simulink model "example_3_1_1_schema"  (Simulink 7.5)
settings: Solver=ode45  StartTime=0.0  StopTime=100  FixedStep=0.001  RelTol=1e-3
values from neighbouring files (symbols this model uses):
  A = [-.4 0 -0.01; 1 0 0; -1.4 9.8 -0.02]    [example_3_1_1_podklad.m]
  AA = A-B*K    [example_3_1_1_podklad.m]
  AAd = Ad-Bd*Kd    [example_3_1_1_podklad.m]
  B = [6.3;0;9.8]    [example_3_1_1_podklad.m]
  C = [0 0 1]    [example_3_1_1_podklad.m]
  D = 0    [example_3_1_1_podklad.m]
  I = eye(m,n)    [example_3_1_1_podklad.m]
  Ng = lqr_kompenzace(A,B,C,D,K)    [example_3_1_1_podklad.m]    (also in lqr_kompenzace.m = Nu + K*Nx)
  T = 0.1    [example_3_1_1_podklad.m]
undefined symbols (not defined in the file or in its folder): Ad, Bd, Cd, Dd, K, Kd

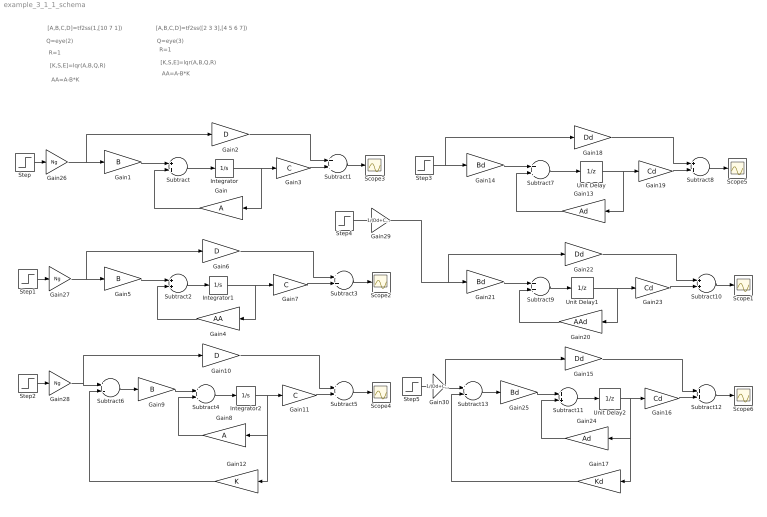
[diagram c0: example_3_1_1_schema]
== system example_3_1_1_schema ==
  note: [A,B,C,D]=tf2ss(1,[10 7 1])
  note: [K,S,E]=lqr(A,B,Q,R)
  note: Q=eye(2)
  note: R=1
  note: [K,S,E]=lqr(A,B,Q,R)
  note: Q=eye(3)
  note: R=1
  note: AA=A-B*K
  note: AA=A-B*K
  note: [A,B,C,D]=tf2ss([2 3 3],[4 5 6 7])
  Gain : Gain  Gain=A  Multiplication=Matrix(K*u)  ParameterDataType=sfix(16)  ParameterScaling=2^0  OutDataType=sfix(16)  OutScaling=2^0
  Gain1 : Gain  Gain=B  Multiplication=Matrix(K*u)  ParameterDataType=sfix(16)  ParameterScaling=2^0  OutDataType=sfix(16)  OutScaling=2^0
  Gain10 : Gain  Gain=D  Multiplication=Matrix(K*u)  ParameterDataType=sfix(16)  ParameterScaling=2^0  OutDataType=sfix(16)  OutScaling=2^0
  Gain11 : Gain  Gain=C  Multiplication=Matrix(K*u)  ParameterDataType=sfix(16)  ParameterScaling=2^0  OutDataType=sfix(16)  OutScaling=2^0
  Gain12 : Gain  Gain=K  Multiplication=Matrix(K*u)  ParameterDataType=sfix(16)  ParameterScaling=2^0  OutDataType=sfix(16)  OutScaling=2^0
  Gain13 : Gain  Gain=Ad  Multiplication=Matrix(K*u)  ParameterDataType=sfix(16)  ParameterScaling=2^0  OutDataType=sfix(16)  OutScaling=2^0
  Gain14 : Gain  Gain=Bd  Multiplication=Matrix(K*u)  ParameterDataType=sfix(16)  ParameterScaling=2^0  OutDataType=sfix(16)  OutScaling=2^0
  Gain15 : Gain  Gain=Dd  Multiplication=Matrix(K*u)  ParameterDataType=sfix(16)  ParameterScaling=2^0  OutDataType=sfix(16)  OutScaling=2^0
  Gain16 : Gain  Gain=Cd  Multiplication=Matrix(K*u)  ParameterDataType=sfix(16)  ParameterScaling=2^0  OutDataType=sfix(16)  OutScaling=2^0
  Gain17 : Gain  Gain=Kd  Multiplication=Matrix(K*u)  ParameterDataType=sfix(16)  ParameterScaling=2^0  OutDataType=sfix(16)  OutScaling=2^0
  Gain18 : Gain  Gain=Dd  Multiplication=Matrix(K*u)  ParameterDataType=sfix(16)  ParameterScaling=2^0  OutDataType=sfix(16)  OutScaling=2^0
  Gain19 : Gain  Gain=Cd  Multiplication=Matrix(K*u)  ParameterDataType=sfix(16)  ParameterScaling=2^0  OutDataType=sfix(16)  OutScaling=2^0
  Gain2 : Gain  Gain=D  Multiplication=Matrix(K*u)  ParameterDataType=sfix(16)  ParameterScaling=2^0  OutDataType=sfix(16)  OutScaling=2^0
  Gain20 : Gain  Gain=AAd  Multiplication=Matrix(K*u)  ParameterDataType=sfix(16)  ParameterScaling=2^0  OutDataType=sfix(16)  OutScaling=2^0
  Gain21 : Gain  Gain=Bd  Multiplication=Matrix(K*u)  ParameterDataType=sfix(16)  ParameterScaling=2^0  OutDataType=sfix(16)  OutScaling=2^0
  Gain22 : Gain  Gain=Dd  Multiplication=Matrix(K*u)  ParameterDataType=sfix(16)  ParameterScaling=2^0  OutDataType=sfix(16)  OutScaling=2^0
  Gain23 : Gain  Gain=Cd  Multiplication=Matrix(K*u)  ParameterDataType=sfix(16)  ParameterScaling=2^0  OutDataType=sfix(16)  OutScaling=2^0
  Gain24 : Gain  Gain=Ad  Multiplication=Matrix(K*u)  ParameterDataType=sfix(16)  ParameterScaling=2^0  OutDataType=sfix(16)  OutScaling=2^0
  Gain25 : Gain  Gain=Bd  Multiplication=Matrix(K*u)  ParameterDataType=sfix(16)  ParameterScaling=2^0  OutDataType=sfix(16)  OutScaling=2^0
  Gain26 : Gain  Gain=Ng  ParameterDataType=sfix(16)  ParameterScaling=2^0  OutDataType=sfix(16)  OutScaling=2^0
  Gain27 : Gain  Gain=Ng  ParameterDataType=sfix(16)  ParameterScaling=2^0  OutDataType=sfix(16)  OutScaling=2^0
  Gain28 : Gain  Gain=Ng  ParameterDataType=sfix(16)  ParameterScaling=2^0  OutDataType=sfix(16)  OutScaling=2^0
  Gain29 : Gain  Gain=1/(Dd+Cd*inv(I-AAd)*Bd)  ParameterDataType=sfix(16)  ParameterScaling=2^0  OutDataType=sfix(16)  OutScaling=2^0
  Gain3 : Gain  Gain=C  Multiplication=Matrix(K*u)  ParameterDataType=sfix(16)  ParameterScaling=2^0  OutDataType=sfix(16)  OutScaling=2^0
  Gain30 : Gain  Gain=1/(Dd+Cd*inv(I-AAd)*Bd)  ParameterDataType=sfix(16)  ParameterScaling=2^0  OutDataType=sfix(16)  OutScaling=2^0
  Gain4 : Gain  Gain=AA  Multiplication=Matrix(K*u)  ParameterDataType=sfix(16)  ParameterScaling=2^0  OutDataType=sfix(16)  OutScaling=2^0
  Gain5 : Gain  Gain=B  Multiplication=Matrix(K*u)  ParameterDataType=sfix(16)  ParameterScaling=2^0  OutDataType=sfix(16)  OutScaling=2^0
  Gain6 : Gain  Gain=D  Multiplication=Matrix(K*u)  ParameterDataType=sfix(16)  ParameterScaling=2^0  OutDataType=sfix(16)  OutScaling=2^0
  Gain7 : Gain  Gain=C  Multiplication=Matrix(K*u)  ParameterDataType=sfix(16)  ParameterScaling=2^0  OutDataType=sfix(16)  OutScaling=2^0
  Gain8 : Gain  Gain=A  Multiplication=Matrix(K*u)  ParameterDataType=sfix(16)  ParameterScaling=2^0  OutDataType=sfix(16)  OutScaling=2^0
  Gain9 : Gain  Gain=B  Multiplication=Matrix(K*u)  ParameterDataType=sfix(16)  ParameterScaling=2^0  OutDataType=sfix(16)  OutScaling=2^0
  Integrator : Integrator
  Integrator1 : Integrator
  Integrator2 : Integrator
  Scope{1..6} (6 alike) : Scope
  Step{,1..5} (6 alike) : Step  Time=0  SampleTime=0
  Subtract{,1..5,7..12} (12 alike) : Sum  OutDataType=sfix(16)  OutScaling=2^-10
  Subtract13 : Sum  Inputs=+-  OutDataType=sfix(16)  OutScaling=2^-10
  Subtract6 : Sum  Inputs=+-  OutDataType=sfix(16)  OutScaling=2^-10
  Unit Delay : UnitDelay  SampleTime=T
  Unit Delay1 : UnitDelay  SampleTime=T
  Unit Delay2 : UnitDelay  SampleTime=T
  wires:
  Integrator/1 -> Gain/1, Gain3/1
  Gain/1 -> Subtract/2
  Subtract/1 -> Integrator/1
  Gain2/1 -> Subtract1/1
  Gain3/1 -> Subtract1/2
  Gain1/1 -> Subtract/1
  Step/1 -> Gain26/1
  Integrator1/1 -> Gain7/1, Gain4/1
  Gain4/1 -> Subtract2/2
  Subtract2/1 -> Integrator1/1
  Gain6/1 -> Subtract3/1
  Gain7/1 -> Subtract3/2
  Gain5/1 -> Subtract2/1
  Step1/1 -> Gain27/1
  Integrator2/1 -> Gain11/1, Gain8/1, Gain12/1
  Gain8/1 -> Subtract4/2
  Subtract4/1 -> Integrator2/1
  Gain10/1 -> Subtract5/1
  Gain11/1 -> Subtract5/2
  Gain9/1 -> Subtract4/1
  Step2/1 -> Gain28/1
  Gain12/1 -> Subtract6/2
  Subtract6/1 -> Gain9/1
  Subtract5/1 -> Scope4/1
  Subtract3/1 -> Scope2/1
  Subtract1/1 -> Scope3/1
  Unit Delay/1 -> Gain19/1, Gain13/1
  Gain13/1 -> Subtract7/2
  Subtract7/1 -> Unit Delay/1
  Gain18/1 -> Subtract8/1
  Gain19/1 -> Subtract8/2
  Gain14/1 -> Subtract7/1
  Step3/1 -> Gain18/1, Gain14/1
  Unit Delay1/1 -> Gain20/1, Gain23/1
  Gain20/1 -> Subtract9/2
  Subtract9/1 -> Unit Delay1/1
  Gain22/1 -> Subtract10/1
  Gain23/1 -> Subtract10/2
  Gain21/1 -> Subtract9/1
  Step4/1 -> Gain29/1
  Unit Delay2/1 -> Gain17/1, Gain24/1, Gain16/1
  Gain24/1 -> Subtract11/2
  Subtract11/1 -> Unit Delay2/1
  Gain15/1 -> Subtract12/1
  Gain16/1 -> Subtract12/2
  Gain25/1 -> Subtract11/1
  Step5/1 -> Gain30/1
  Gain17/1 -> Subtract13/2
  Subtract13/1 -> Gain25/1
  Subtract12/1 -> Scope6/1
  Subtract10/1 -> Scope1/1
  Subtract8/1 -> Scope5/1
  Gain26/1 -> Gain1/1, Gain2/1
  Gain27/1 -> Gain6/1, Gain5/1
  Gain28/1 -> Subtract6/1, Gain10/1
  Gain29/1 -> Gain21/1, Gain22/1
  Gain30/1 -> Gain15/1, Subtract13/1
